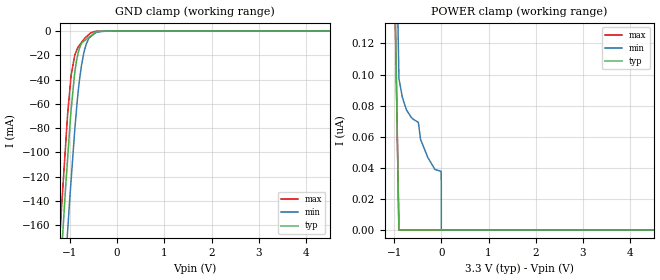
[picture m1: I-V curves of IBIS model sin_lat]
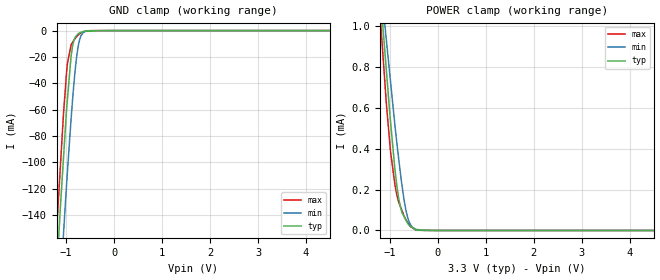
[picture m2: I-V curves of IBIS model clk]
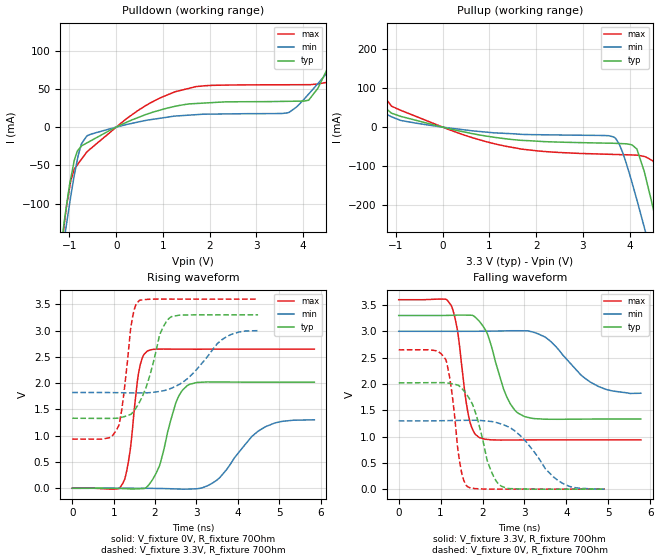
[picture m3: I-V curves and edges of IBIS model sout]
|Texas Instruments Incorporated
| 16-Channel, 12-Bit ES-PWM, Full Self-Diagnosis LED Driver with 7-Bit Global
| BC LED Lamp
| Marketing part#   Digital Voltage Range   Package-type   #pins
| TLC5949DBQ   3.0V-3.6V   SSOP   24
| TLC5949DBQR   3.0V-3.6V   SSOP   24
| TLC5949PWP   3.0V-3.6V   HTSSOP   24
| TLC5949PWPR   3.0V-3.6V   HTSSOP   24
[IBIS Ver]   3.2
[File name]   tlc5949.ibs
[File Rev]   1.0
[Date]   12/14/2012
[Source]
| Texas Instruments Incorporated.
| Analog-eLab Design Center, HPA
| 12500 TI Blvd
| Dallas, TX -75243
| e-mail: elab_scm_ibis@list.ti.com
[Notes]   Revision History:
| Rev 1.0: 12/14/2012
| - Initial version of the model
| - Model generated from simulations in TISPICE
| - Model matched to SPICE simulation
| - C_comp although listed in numerical order of value are
|   obtained from varying PVT conditions. For PVT conditions for
|   each specific value refer the buffer description under
|   respective [Model]. IBIS model user is responsible for using
|   appropriate C_comp to simulate for Signal Integrity.
| - Model names with a trailing _3p3 contains the model for
|   3.3V [3.0V and 3.6V].
[Disclaimer]
| This model is designed as an aid for customers of Texas Instruments.
| TI and its licensors and suppliers make no warranties, either expressed
| or implied, with respect to this  model, including the warranties of
| merchantability or fitness for a particular purpose. The model is
| provided solely on an "as is" basis. The entire risk as to its quality
| and performance is with the customer.
[Copyright]
(C) Copyright 2012 Texas Instruments Incorporated.All rights reserved.
|   TLC5949DBQ
[Component]   TLC5949DBQ
[Manufacturer]   TI
[Package]   |24 SSOP   -  DBQ package
|   typ   min   max
R_pkg   0.10367   0.06399   0.13778
L_pkg   2.98041nH   2.00949nH   4.28150nH
C_pkg   0.44498pF   0.36340pF   0.58072pF
[Pin]  signal_name   model_name   R_pin   L_pin   C_pin
1   GND   gnd   0.03881   4.53088nH  0.76812pF
2   SIN   sin_lat   0.11731   3.63731nH  0.55194pF
3   SCLK   clk   0.10472   2.82203nH  0.41499pF
4   LAT   sin_lat   0.07611   2.22754nH  0.37434pF
5   OUT0   term   0.09994   2.66697nH  0.39651pF
6   OUT1   term   0.09397   2.55648nH  0.39270pF
7   OUT2   term   0.09614   2.59848nH  0.39590pF
8   OUT3   term   0.10586   2.78215nH  0.40611pF
9   OUT4   term   0.12161   3.08254nH  0.42406pF
10   OUT5   term   0.13778   3.45793nH  0.44927pF
11   OUT6   term   0.13663   4.01728nH  0.57443pF
12   OUT7   term   0.12288   4.28150nH  0.57999pF
13   OUT8   term   0.12165   4.25808nH  0.58072pF
14   OUT9   term   0.12915   3.87444nH  0.56968pF
15   OUT10   term   0.12129   3.14368nH  0.43664pF
16   OUT11   term   0.10092   2.69263nH  0.40658pF
17   OUT12   term   0.08146   2.32931nH  0.38287pF
18   OUT13   term   0.06742   2.07276nH  0.36756pF
19   OUT14   term   0.06399   2.00949nH  0.36340pF
20   OUT15   term   0.07312   2.17191nH  0.37095pF
21   GSCLK   clk   0.09130   2.50639nH  0.39119pF
22   SOUT   sout   0.09999   2.73316nH  0.40875pF
23   IREF   term   0.11759   3.64697nH  0.55090pF
24   VCC   power   0.11604   4.14665nH  0.56614pF
|   TLC5949PWP
[Component]   TLC5949PWP
[Manufacturer]   TI
[Package]   |24 HTSSOP -  PWP package
|   typ   min   max
R_pkg   0.24801   0.18592   0.33621
L_pkg   1.96166nH   1.43721nH   2.82419nH
C_pkg   0.29977pF   0.23581pF   0.40028pF
[Pin]  signal_name   model_name   R_pin   L_pin   C_pin
1   GND   gnd   0.09474   1.90076nH  0.57180pF
2   SIN   sin_lat   0.23981   1.90618nH  0.31487pF
3   SCLK   clk   0.24221   1.88219nH  0.25796pF
4   LAT   sin_lat   0.20264   1.55349nH  0.25681pF
5   OUT0   term   0.26394   2.06242nH  0.25727pF
6   OUT1   term   0.25237   1.96674nH  0.25465pF
7   OUT2   term   0.25682   2.00384nH  0.27877pF
8   OUT3   term   0.27627   2.16968nH  0.26811pF
9   OUT4   term   0.31448   2.53437nH  0.34002pF
10   OUT5   term   0.33621   2.82419nH  0.40028pF
11   OUT6   term   0.30214   2.53832nH  0.38760pF
12   OUT7   term   0.25435   2.03198nH  0.31498pF
13   OUT8   term   0.22900   1.77747nH  0.24960pF
14   OUT9   term   0.25336   1.97693nH  0.28138pF
15   OUT10   term   0.27769   2.18075nH  0.27150pF
16   OUT11   term   0.25692   2.00711nH  0.26110pF
17   OUT12   term   0.21524   1.66000nH  0.26321pF
18   OUT13   term   0.18783   1.43721nH  0.23581pF
19   OUT14   term   0.18592   1.46560nH  0.29001pF
20   OUT15   term   0.21275   1.79248nH  0.34832pF
21   GSCLK   clk   0.23511   1.82095nH  0.35508pF
22   SOUT   sout   0.22714   1.75446nH  0.35174pF
23   IREF   term   0.23393   1.81016nH  0.35593pF
24   VCC   power   0.22320   1.72139nH  0.34977pF
[Model] term
Model_type Terminator
C_comp   1.0e-20F  1.0e-20F  1.0e-20F
|   typ   min   max
[Voltage Range]   3.3V   3.0V   3.6V
[POWER Clamp Reference]   3.3V   3.0V   3.6V
[GND Clamp Reference]   0V   0V   0V
|Ambient Temperature   25   85   -40
|Junction Temperature
[Temperature Range]   27   125   -40
| Models and submodels in the file (4): sin_lat (Input), clk (Input), sout (Output), term (Terminator)
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|   sin_lat Model
[Model]   sin_lat
Model_type   Input
Vinl = 0.99
Vinh = 2.31
|   typ   min   max
|   (nom PVT)   (fast PVT)   (slow PVT)
|C_comp from frequency sweep method (F=16.5 MHz)
|Average
|C_comp   2.958e-12   2.743e-12   3.183e-12
|C_comp from LC tank measurement(L=1nH)
|Average
|Resonant Frequency(Hz)   4.030e+09   4.110e+09   3.900e+09
 C_comp   1.561e-12   1.501e-12   1.667e-12
| Where nom  PVT is Nominal Process, 3.3V, 27C
|   Fast PVT is Strong Process,  3.6V, -40C
|   Slow PVT is Weak Process,   3V, 125C
[Voltage Range]   3.3   3   3.6
|Ambient Temperature   25   85   -40
|Junction Temperature
[Temperature Range]   27   125   -40
[Power Clamp Reference]   3.3   3   3.6
[GND Clamp Reference]   0   0   0
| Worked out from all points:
|   GND clamp passes 1 mA (typ) near -0.46 V on its own axis
[GND Clamp]
|   Voltage   I(typ)   I(min)   I(max)
-3.3V     -1.656A    -1.675A    -1.654A
-1.27V    -241.9mA   -302.3mA   -207.8mA
-1.174V   -180.9mA   -241mA     -143.6mA
-1.146V   -163.6mA   -223.6mA   -127.1mA
-1.048V   -104.9mA   -164.6mA   -68.41mA
-975.6mV  -65.57mA   -123.8mA   -37.07mA
-897.6mV  -34.22mA   -81.91mA   -19.82mA
-801mV    -14.71mA   -41.57mA   -11.91mA
-702mV    -8.284mA   -17.47mA   -6.652mA
-561.6mV  -4.041mA   -4.643mA   -1.501mA
-201mV    -123.2uA   -10.18uA   -16.14uA
6.6V      0A         0A         0A
[POWER Clamp]
|   Voltage   I(typ)   I(min)   I(max)
-3.3V     55.85uA    44.07uA    72.09uA
-1.365V   837.4nA    872nA      825.2nA
-897.6mV  0A         98.45nA    0A
-825mV    0A         85.43nA    0A
-741mV    0A         77.5nA     0A
-486mV    0A         69.28nA    0A
-439.2mV  0A         58.39nA    0A
-285mV    0A         46.63nA    0A
-3mV      0A         37.75nA    0A
-33.83fV  0A         29.07nA    0A
0V        0A         0A         0A
6.6V      0A         0A         0A
|   clk Model
[Model]   clk
Model_type   Input
Vinl = 0.99
Vinh = 2.31
|   typ   min   max
|   (nom PVT)   (fast PVT)   (slow PVT)
|C_comp from frequency sweep method (F=33MHz)
|Average
|C_comp   8.187e-13   7.978e-13   8.482e-13
|C_comp from LC tank measurement(L=1nH)
|Average
|Resonant Frequency(Hz)   6.700e+09   6.850e+09   6.560e+09
 C_comp   5.648e-13   5.404e-13   5.892e-13
| Where nom  PVT is Nominal Process, 3.3V, 27C
|   Fast PVT is Strong Process,  3.6V, -40C
|   Slow PVT is Weak Process,   3V, 125C
[Voltage Range]   3.3   3   3.6
|Ambient Temperature   25   85   -40
|Junction Temperature
[Temperature Range]   27   125   -40
[Power Clamp Reference]   3.3   3   3.6
[GND Clamp Reference]   0   0   0
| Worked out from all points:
|   GND clamp passes 1 mA (typ) near -0.66 V on its own axis
|   POWER clamp passes 1 mA (typ) near -1.15 V on its own axis
[GND Clamp]
|   Voltage   I(typ)   I(min)   I(max)
-3.3V     -1.684A    -1.679A    -1.716A
-1.202V   -187.4mA   -244.7mA   -155.6mA
-1.167V   -164.6mA   -222.1mA   -132.4mA
-1.122V   -135.6mA   -194.5mA   -104.7mA
-1.055V   -96.76mA   -154.6mA   -63.39mA
-972mV    -51.72mA   -106.8mA   -24.75mA
-897.6mV  -19.78mA   -67.62mA   -11.05mA
-838.2mV  -7.497mA   -40.69mA   -7.349mA
-786mV    -3.891mA   -21.48mA   -4.862mA
-693mV    -1.291mA   -4.142mA   -1.915mA
-285mV    -110.1uA   -2.527uA   -7.129uA
6.6V      0A         0A         0A
[POWER Clamp]
|   Voltage   I(typ)   I(min)   I(max)
-3.3V     8.146mA    6.63mA     9.069mA
-1.213V   1.208mA    1.258mA    1.087mA
-1.142V   984.9uA    1.091mA    848.6uA
-1.076V   792.5uA    938.3uA    630.4uA
-986.4mV  532.1uA    728.1uA    386.6uA
-897.6mV  305.3uA    520.7uA    228.1uA
-821.7mV  164.8uA    360.7uA    142.5uA
-714mV    72.64uA    164.5uA    76.74uA
-627mV    33.96uA    60.96uA    38.39uA
-534mV    15.01uA    16.71uA    13.38uA
-453.6mV  2.741uA    5.423uA    1.489uA
6.6V      0A         0A         0A
|   sout Model
[Model]   sout
Model_type   Output
Polarity   Non-Inverting
Vmeas = 1.65
Vref = 1.65
Cref = 15pF
Rref = 50
|   typ   min   max
|   (nom PVT)   (fast PVT)   (slow PVT)
|C_comp from frequency sweep method (F=16.5 MHz)
|C_comp   1.965e-12   1.934e-12   2.050e-12
|ON state : BUFFER OUTPUT TURNED HIGH
|C_comp   1.965e-12   1.934e-12   2.050e-12
|OFF state: BUFFER OUTPUT TURNED LOW
|C_comp   2.320e-12   2.234e-12   2.465e-12
|C_comp from LC tank measurement(L=1nH)
|Resonant Frequency(Hz)   4.460e+09   4.580e+09   4.230e+09
 C_comp   1.275e-12   1.209e-12   1.417e-12
|ON state : BUFFER OUTPUT TURNED HIGH
|Resonant Frequency(Hz)   4.460e+09   4.580e+09   4.230e+09
|C_comp   1.275e-12   1.209e-12   1.417e-12
|OFF state: BUFFER OUTPUT TURNED LOW
|Resonant Frequency(Hz)   4.320e+09   4.450e+09   4.130e+09
|C_comp   1.359e-12   1.280e-12   1.487e-12
| Where nom  PVT is Nominal Process, 3.3V, 27C
|   Fast PVT is Strong Process,  3.6V, -40C
|   Slow PVT is Weak Process,   3V, 125C
[Voltage Range]   3.3   3   3.6
|Ambient Temperature   25   85   -40
|Junction Temperature
[Temperature Range]   27   125   -40
[Pullup Reference]   3.3   3   3.6
[Pulldown Reference]   0   0   0
[Power Clamp Reference]   3.3   3   3.6
[GND Clamp Reference]   0   0   0
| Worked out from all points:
|   slope of the pulldown table from 0 to 0.495 V, typ, clamps not added: 37.5 ohm
|   slope of the pullup table from 0 to 0.495 V, typ, clamps not added: 37.5 ohm
|   falling waveform, V_fixture 3.3V, R_fixture 70Ohm: 20-80 % time 460ps typ, 851ps min, 258ps max; typ from 3.3 V to 1.33 V
|   rising waveform, V_fixture 0V, R_fixture 70Ohm: 20-80 % time 404ps typ, 798ps min, 226ps max; typ from 0 V to 2.02 V
|   rising waveform, V_fixture 3.3V, R_fixture 70Ohm: 20-80 % time 427ps typ, 785ps min, 228ps max; typ from 1.33 V to 3.3 V
|   falling waveform, V_fixture 0V, R_fixture 70Ohm: 20-80 % time 418ps typ, 787ps min, 237ps max; typ from 2.02 V to 0 V
[Pulldown]
|   Voltage   I(typ)   I(min)   I(max)
-3.3V     -1.356A    -1.19A     -1.685A
-1.105V   -120.1mA   -143.9mA   -123.6mA
-897.6mV  -43.25mA   -62.75mA   -54.89mA
-744mV    -24.51mA   -21.76mA   -41.92mA
-630mV    -20.69mA   -11.58mA   -32.4mA
1.267V    27.31mA    14.49mA    46.32mA
3.669V    33.7mA     18.66mA    55.34mA
4.118V    35.12mA    43.18mA    55.42mA
4.507V    74.86mA    70.4mA     58.63mA
4.709V    101.6mA    84.9mA     92.61mA
5.864V    254.7mA    168mA      424.2mA
6.6V      352.2mA    220.9mA    597.5mA
[Pullup]
|   Voltage   I(typ)   I(min)   I(max)
-3.3V     319mA      181.6mA    601.6mA
-2.84V    258.9mA    148.9mA    508.2mA
-1.994V   148.1mA    88.67mA    296.7mA
-1.096V   35.66mA    26.37mA    53.59mA
1.246V    -28.16mA   -15.4mA    -46.22mA
3.66V     -41.18mA   -25mA      -69.73mA
3.855V    -42.21mA   -65.68mA   -70.36mA
4.158V    -56.27mA   -186.4mA   -71.56mA
4.316V    -114mA     -256.6mA   -74.97mA
4.554V    -233.3mA   -365.5mA   -98.23mA
4.795V    -364.1mA   -480mA     -242.7mA
6.6V      -1.401A    -1.362A    -1.557A
[Ramp]
R_load = 70
|   typ   min   max
dV/dt_r   1.22818/3.98594e-10   0.795642/7.82521e-10   1.60228/2.23931e-10
dV/dt_f   1.19846/4.54148e-10   0.72397/8.45599e-10   1.61321/2.54808e-10
[Falling Waveform]
V_fixture = 3.3V
V_fixture_min = 3V
V_fixture_max = 3.6V
R_fixture = 70Ohm
C_fixture = 0F
|   Time   V(typ)   V(min)   V(max)
0s        3.3V       3V         3.6V
1.25ns    3.304V     3V         3.492V
1.4ns     3.308V     2.999V     3.03V
1.67ns    3.306V     3V         1.382V
1.93ns    3.185V     3.001V     979.5mV
2.58ns    1.752V     3.009V     933.1mV
2.86ns    1.439V     3.01V      934.4mV
3.51ns    1.329V     2.882V     935.8mV
4.78ns    1.332V     1.947V     935.9mV
5.779ns   1.333V     1.823V     935.8mV
[Rising Waveform]
V_fixture = 0V
V_fixture_min = 0V
V_fixture_max = 0V
R_fixture = 70Ohm
C_fixture = 0F
|   Time   V(typ)   V(min)   V(max)
0s        1.372nV    9.021nV    965.1pV
1.22ns    -5.43mV    529.2uV    93.15mV
1.39ns    -11.96mV   625uV      671.8mV
1.61ns    -9.996mV   93.18uV    2.225V
1.82ns    39.36mV    -894.8uV   2.614V
2.5ns     1.621V     -12.08mV   2.648V
2.78ns    1.954V     -15.92mV   2.647V
3.5ns     2.024V     157.3mV    2.647V
4.67ns    2.019V     1.172V     2.647V
5.85ns    2.019V     1.303V     2.647V
[Rising Waveform]
V_fixture = 3.3V
V_fixture_min = 3V
V_fixture_max = 3.6V
R_fixture = 70Ohm
C_fixture = 0F
|   Time   V(typ)   V(min)   V(max)
0s        1.333V     1.823V     935.9mV
870ps     1.33V      1.822V     957.8mV
1.12ns    1.339V     1.819V     1.187V
1.24ns    1.36V      1.818V     1.761V
1.44ns    1.425V     1.815V     3.178V
1.62ns    1.633V     1.815V     3.573V
2.11ns    2.915V     1.843V     3.601V
2.37ns    3.253V     1.896V     3.6V
3.63ns    3.3V       2.835V     3.6V
4.49ns    3.3V       3V         3.6V
[Falling Waveform]
V_fixture = 0V
V_fixture_min = 0V
V_fixture_max = 0V
R_fixture = 70Ohm
C_fixture = 0F
|   Time   V(typ)   V(min)   V(max)
0s        2.019V     1.297V     2.647V
1.13ns    2.02V      1.301V     2.451V
1.27ns    2.003V     1.303V     1.831V
1.46ns    1.95V      1.306V     495.1mV
1.64ns    1.778V     1.308V     46.97mV
1.85ns    1.408V     1.308V     8.673mV
2.12ns    525.1mV    1.293V     462.4uV
2.41ns    76.86mV    1.247V     -599.9uV
3.83ns    -500.7uV   148.6mV    23.9uV
4.92ns    2.252uV    7.676uV    4.679nV
